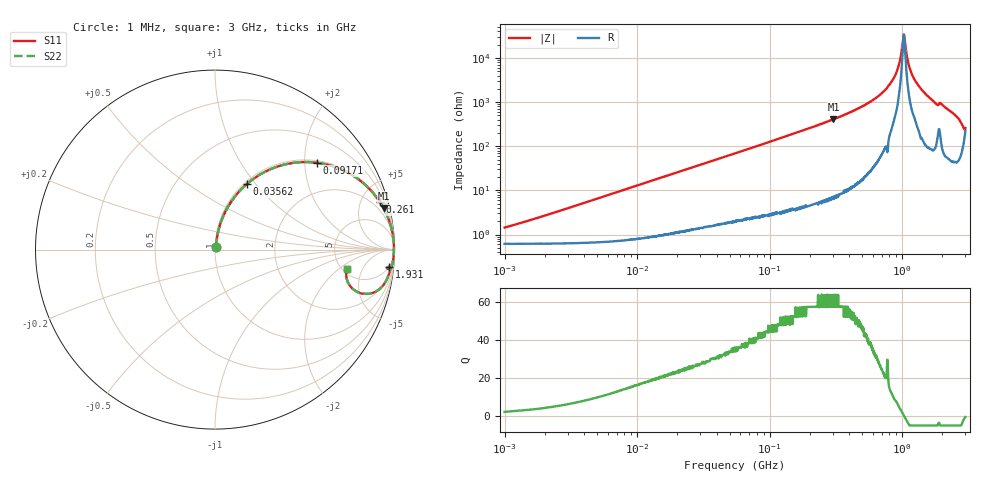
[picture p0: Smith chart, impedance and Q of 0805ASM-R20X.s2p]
!s-Parameter Generated by FASTRON Sdn. Bhd.
!FASTRON P/N : 0805ASM-R20X
!Keysight Technologies: E4991B_MY54100416_A.01.15
!Date: Fri Jun 19 14:50:57 2026
!Version  :Rev00  Fri Jun 19 14:50:57 2026
!Data & Calibration Information:
!Freq  S11  S21  S12  S22
!PortZ  Port1:50+j0  Port2:50+j0
!When reading reference impedance value at option line is always used.
! Remarks : This data is being provided solely for informational purposes.
# Hz S dB R 50
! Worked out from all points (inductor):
!   1601 points, 1 MHz to 3 GHz, reference 50 ohm
!   read as one part in series: L = 207 nH near 1.427 MHz
!   highest Q = 63.6 at 303.2 MHz (marker M1), where L = 214 nH
!   self-resonance near 1.028 GHz
!   S11 on the Smith chart (normalised r, x): 1 MHz: 1.01, +0.03; 35.62 MHz: 1.03, +0.90; 91.71 MHz: 1.05, +2.31; 261 MHz: 1.12, +6.89; 1.931 GHz: 5, -19; 3 GHz: 5.49, -2.60
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1000000  -36.90 64.0  -0.05 -0.7  -0.05 -0.7  -36.90 64.0
3804036  -26.10 79.8  -0.07 -2.8  -0.07 -2.8  -26.10 79.8
1.447069e7  -14.80 76.7  -0.23 -10.4  -0.23 -10.4  -14.80 76.7
3.561766e7  -7.83 64.1  -0.92 -24.0  -0.92 -24.0  -7.83 64.1
5.504702e7  -5.00 54.1  -1.82 -34.2  -1.82 -34.2  -5.00 54.1
9.170654e7  -2.53 40.3  -3.77 -48.3  -3.77 -48.3  -2.53 40.3
2.083556e8  -0.61 20.3  -9.20 -68.7  -9.20 -68.7  -0.61 20.3
2.609752e8  -0.39 16.1  -11.10 -72.9  -11.10 -72.9  -0.39 16.1
3.032461e8  -0.29 13.7  -12.50 -75.4  -12.50 -75.4  -0.29 13.7
5.63991e8  -0.07 5.8  -19.90 -82.7  -19.90 -82.7  -0.07 5.8
7.925923e8  -0.03 2.4  -27.60 -84.1  -27.60 -84.1  -0.03 2.4
9.117997e8  -0.03 1.1  -34.00 -80.7  -34.00 -80.7  -0.03 1.1
9.538021e8  -0.03 0.7  -37.90 -76.4  -37.90 -76.4  -0.03 0.7
1.002744e9  -0.03 0.3  -45.60 -56.5  -45.60 -56.5  -0.03 0.3
1.033307e9  -0.03 -0.0  -50.60 9.2  -50.60 9.2  -0.03 -0.0
1.142072e9  -0.03 -1.0  -35.30 78.2  -35.30 78.2  -0.03 -1.0
1.249715e9  -0.04 -1.8  -29.90 80.8  -29.90 80.8  -0.04 -1.8
1.565327e9  -0.07 -4.2  -22.70 81.9  -22.70 81.9  -0.07 -4.2
1.931433e9  -0.22 -5.7  -19.90 72.7  -19.90 72.7  -0.22 -5.7
2.620866e9  -0.40 -12.3  -13.40 71.9  -13.40 71.9  -0.40 -12.3
2.825159e9  -0.97 -16.0  -11.00 60.3  -11.00 60.3  -0.97 -16.0
3e9  -2.59 -8.3  -10.90 21.9  -10.90 21.9  -2.59 -8.3
